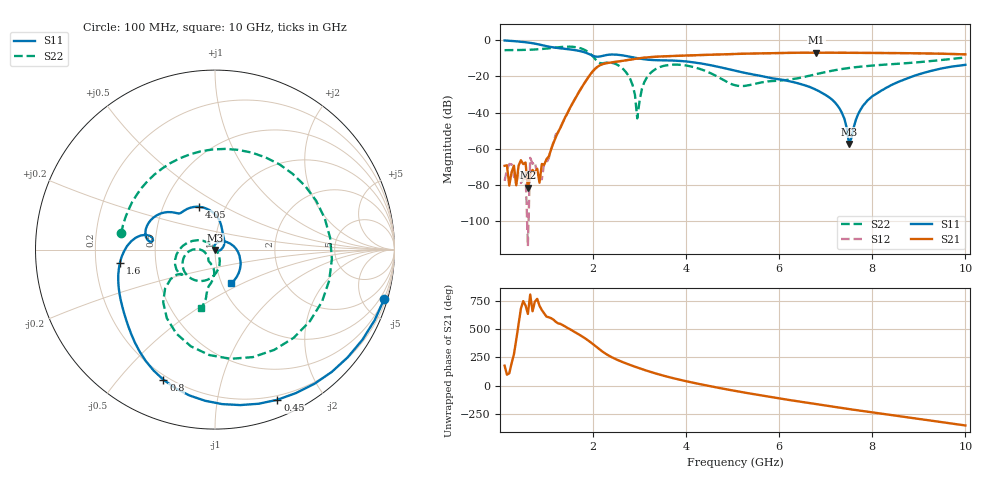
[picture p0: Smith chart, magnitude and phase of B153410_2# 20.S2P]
!  2-Port S-parameters saved by WinCal
! VAR MeasName=S-Parameters (CALIBRATED_DATA) read from VNA (N5245A)
! VAR MeasDate=2016-12-23 10:00:21
! VAR NAME=B153410_2# 20
! VAR FILENAME=B153410_2# 20.S2P
! VAR DATE=2016-12-23 10:00:21
! VAR PHYS_PORTS=1,2
# Hz S DB R 50
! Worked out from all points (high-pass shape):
!   199 points, 100 MHz to 10 GHz, reference 50 ohm
!   highest |S21| = -6.90 dB at 6.8 GHz (marker M1); lowest = -81.5 dB at 600 MHz (marker M2)
!   |S21| within 3 dB of the highest: 3.021 GHz to end of sweep
!   lowest |S11| = -57.3 dB at 7.5 GHz (marker M3), VSWR 1.00, Z = 50 - j0.137 ohm
!   |S11| at or under -10 dB: 2.964 GHz to end of sweep
!   |S22| runs from -43.2 to -3.6 dB; largest |S21 - S12| = 0.0031
!   S11 on the Smith chart (normalised r, x): 100 MHz: 0.45, -7.01; 450 MHz: 0.16, -1.49; 800 MHz: 0.18, -0.66; 1.6 GHz: 0.30, -0.06; 4.05 GHz: 0.75, +0.38; 10 GHz: 1.11, -0.44
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1e8  -0.15 -16.2  -69.38 177.4  -77.70 -61.4  -5.51 170.2
2.5e8  -0.43 -39.0  -72.92 -161.3  -68.60 59.1  -5.51 155.4
3.5e8  -0.62 -53.4  -80.15 47.5  -79.49 142.3  -5.47 145.0
4.5e8  -0.86 -67.4  -66.31 -36.1  -78.90 16.7  -5.42 134.4
6e8  -1.29 -87.4  -81.54 -83.2  -113.78 57.7  -5.32 117.2
6.5e8  -1.47 -93.7  -74.27 88.7  -65.00 172.0  -5.27 111.1
8e8  -2.16 -111.6  -70.99 50.2  -74.20 -64.4  -5.07 91.5
8.5e8  -2.44 -117.0  -78.73 -12.0  -74.16 -23.0  -4.98 84.4
1.6e9  -5.44 -172.1  -32.94 119.0  -33.00 118.6  -3.76 -59.4
1.75e9  -6.19 177.6  -26.34 81.1  -26.39 80.9  -4.61 -93.0
2.7e9  -8.68 147.4  -11.14 -161.2  -11.14 -161.3  -17.42 159.0
2.95e9  -9.94 139.1  -10.15 161.1  -10.15 160.8  -43.18 80.0
3.1e9  -10.55 136.7  -9.66 140.0  -9.68 139.8  -23.28 -66.9
3.4e9  -11.09 132.4  -9.07 101.7  -9.08 101.6  -15.25 -103.7
4.05e9  -11.87 110.5  -8.45 35.1  -8.46 35.0  -14.23 -158.4
5.05e9  -16.83 76.7  -7.60 -46.3  -7.62 -46.2  -24.89 -161.9
6.7e9  -26.32 18.4  -6.90 -158.6  -6.93 -158.5  -19.33 -93.8
6.8e9  -27.49 11.8  -6.90 -165.0  -6.93 -164.8  -18.71 -92.7
7.3e9  -37.87 -27.6  -6.94 164.2  -6.95 164.3  -16.10 -93.1
7.5e9  -57.26 -92.5  -6.96 152.3  -6.99 152.3  -15.35 -94.6
8.35e9  -25.64 57.9  -7.12 102.4  -7.12 102.6  -13.37 -100.2
1e10  -13.61 -64.1  -7.83 6.9  -7.84 7.3  -9.54 -103.1
